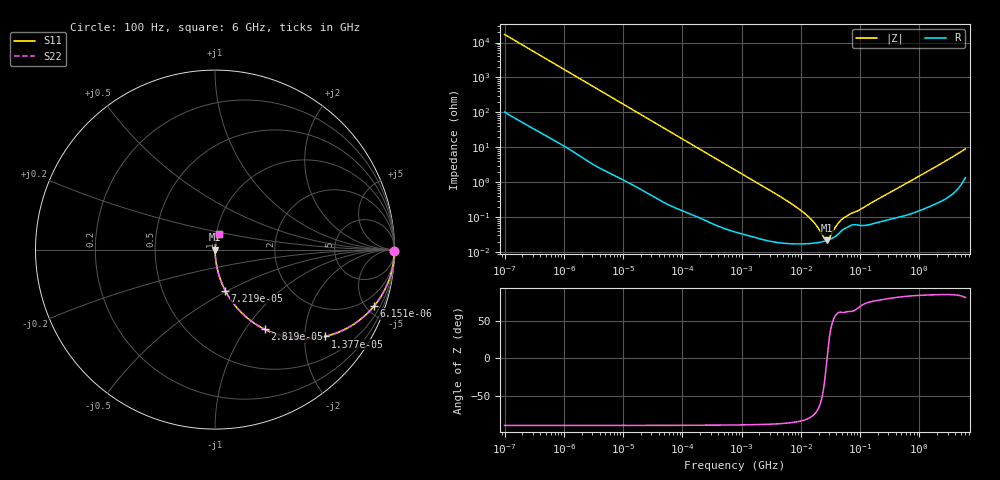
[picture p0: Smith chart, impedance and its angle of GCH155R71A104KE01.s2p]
!Murata Part Number: GCH155R71A104KE01
!These Parameters are Measured in Series Mode Connection
!Data Generated on Mar 13, 2026
!  o--ll--o
!Port1  Port2
!  o------o
!Operation Temp=25[degC], DC Bias Voltage=0[V]
!Freq. Start=100[Hz] Stop=6[GHz] 401[Steps]
# Hz S RI R 50
!Freq.(Hz) S11(Real) S11(Imag) S21(Real) S21(Imag) S12(Real) S12(Imag) S22(Real) S22(Imag)
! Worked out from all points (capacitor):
!   401 points, 100 Hz to 6 GHz, reference 50 ohm
!   read as one part in series: C = 93.3 nF near 109 Hz
!   lowest |Z| = 21.7 mohm at 27.84 MHz (marker M1)
!   series resonance near 27.64 MHz, so ESL is about 360 pH
!   S11 on the Smith chart (normalised r, x): 100 Hz: open; 6.151 kHz: 1.04, -5.63; 13.77 kHz: 1.02, -2.52; 28.19 kHz: 1.01, -1.24; 72.19 kHz: 1.00, -0.48; 6 GHz: 1.03, +0.18
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100  0.9999 -0.00587  6.96e-05 0.00587  6.96e-05 0.00587  0.9999 -0.00587
627  0.9984 -0.0365  0.00156 0.0365  0.00156 0.0365  0.9984 -0.0365
2008  0.9859 -0.1148  0.0141 0.1148  0.0141 0.1148  0.9859 -0.1148
6151  0.8863 -0.3143  0.1137 0.3143  0.1137 0.3143  0.8863 -0.3143
9204  0.7785 -0.4119  0.2215 0.4119  0.2215 0.4119  0.7785 -0.4119
13772  0.6131 -0.4836  0.3869 0.4836  0.3869 0.4836  0.6131 -0.4836
28191  0.2778 -0.4443  0.7222 0.4443  0.7222 0.4443  0.2778 -0.4443
40335  0.1595 -0.3625  0.8405 0.3625  0.8405 0.3625  0.1595 -0.3625
72189  0.057 -0.228  0.943 0.228  0.943 0.228  0.057 -0.228
193316  0.00914 -0.09  0.9909 0.09  0.9909 0.09  0.00914 -0.09
774597  0.000899 -0.0228  0.9991 0.0228  0.9991 0.0228  0.000899 -0.0228
6644369  0.00018 -0.00255  0.9998 0.00255  0.9998 0.00255  0.00018 -0.00255
1.087309e7  0.000174 -0.0014  0.9998 0.0014  0.9998 0.0014  0.000174 -0.0014
1.555665e7  0.000179 -0.00079  0.9998 0.00079  0.9998 0.00079  0.000179 -0.00079
1.946e7  0.000188 -0.000466  0.9998 0.000466  0.9998 0.000466  0.000188 -0.000466
2.434276e7  0.000203 -0.000166  0.9998 0.000166  0.9998 0.000166  0.000203 -0.000166
2.784235e7  0.000217 9.6e-06  0.9998 -9.6e-06  0.9998 -9.6e-06  0.000217 9.6e-06
3.045065e7  0.000229 0.000127  0.9998 -0.000127  0.9998 -0.000127  0.000229 0.000127
4.165952e7  0.000313 0.00055  0.9997 -0.00055  0.9997 -0.00055  0.000313 0.00055
5.211241e7  0.00045 0.000816  0.9996 -0.000816  0.9996 -0.000816  0.00045 0.000816
3.124326e8  0.000883 0.0049  0.9991 -0.0049  0.9991 -0.0049  0.000883 0.0049
6e9  0.021 0.0863  0.979 -0.0863  0.979 -0.0863  0.021 0.0863
